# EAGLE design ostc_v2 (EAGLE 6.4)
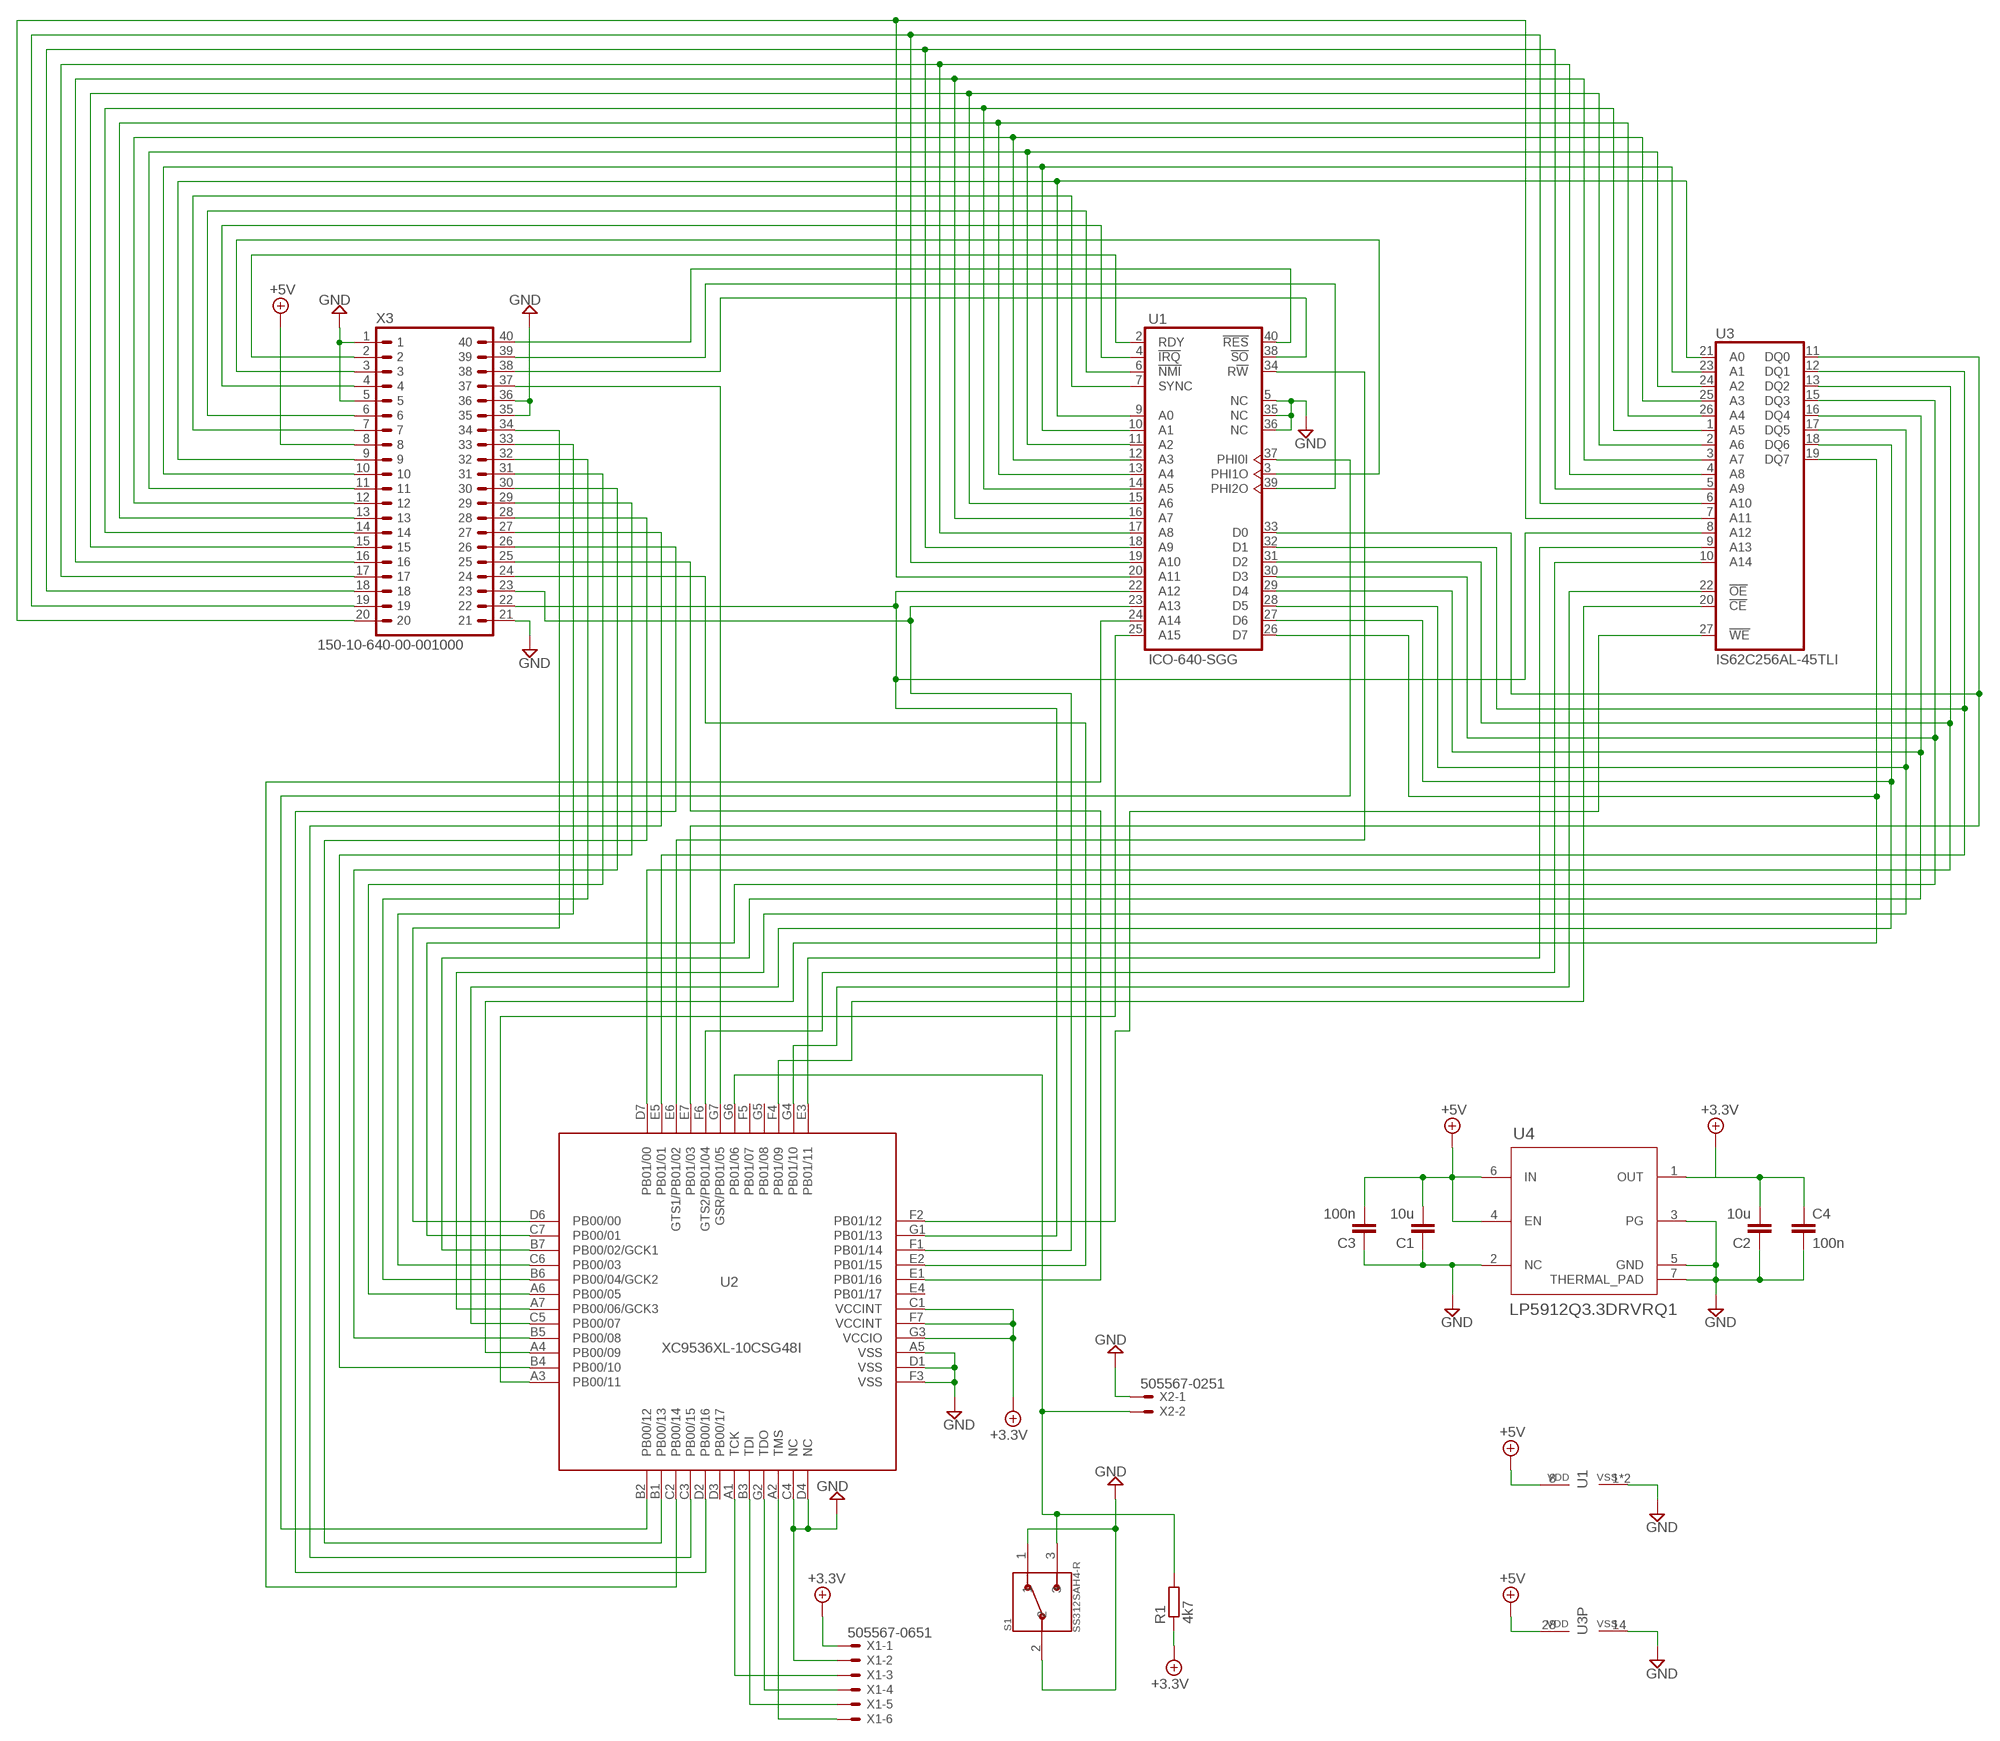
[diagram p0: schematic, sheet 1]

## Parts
C1  10u  C-EUC1206K  [C1206K]
C2  10u  C-EUC1206K  [C1206K]
C3  100n  C-EUC1206K  [C1206K]
C4  100n  C-EUC1206K  [C1206K]
R1  4k7  R-EU_R0805  [R0805]
S1  SS312SAH4-R  [SW_SS312SAH4-R]
U1  ICO-640-SGG  6502  [DIL40_LOWPROFILE]
U2  XC9536XL-10CSG48I  CX9536_CS48  [CSBGA48]
U3  IS62C256AL-45TLI  CY62256LL-ZC  [TSOP1-28]
U4  LP5912Q3.3DRVRQ1  LP5912-3.0DRVT  [DRV0006A-IPC_A]
X1  505567-0651  53261-06  [53261-06]
X2  505567-0251  53261-02  [53261-02]
X3  150-10-640-00-001000  DIL40  [DIL40]

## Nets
+3.3V: C2.2 C4.1 R1.1 U2.C1(VCCINT) U2.F7(VCCINT) U2.G3(VCCIO) U4.1(OUT) X1.1
+5V: C1.2 C3.2 U1.8(VDD) U3.28(VDD) U4.4(EN) U4.6(IN) X3.8
GND: C1.1 C2.1 C3.1 C4.2 S1.1 S1.2 U1.1(VSS) U1.5(NC) U1.21(VSS) U1.35(NC) U1.36(NC) U2.A5(VSS) U2.C4(NC) U2.D1(VSS) U2.D4(NC) U2.F3(VSS) U3.14(VSS) U4.2(NC) U4.3(PG) U4.5(GND) U4.7(THERMAL_PAD) X1.2 X2.1 X3.1 X3.5 X3.21 X3.35 X3.36
N$1: U1.2(RDY) X3.2
N$2: U1.3(PHI1O) X3.3
N$3: U1.4(!IRQ) X3.4
N$4: U1.6(!NMI) X3.6
N$5: U1.7(SYNC) X3.7
N$6: U1.9(A0) U3.21(A0) X3.9
N$7: U1.10(A1) U3.23(A1) X3.10
N$8: U1.11(A2) U3.24(A2) X3.11
N$9: U1.12(A3) U3.25(A3) X3.12
N$10: U1.13(A4) U3.26(A4) X3.13
N$11: U1.14(A5) U3.1(A5) X3.14
N$12: U1.15(A6) U3.2(A6) X3.15
N$13: U1.16(A7) U3.3(A7) X3.16
N$14: U1.17(A8) U3.4(A8) X3.17
N$15: U1.18(A9) U3.5(A9) X3.18
N$16: U1.19(A10) U3.6(A10) X3.19
N$17: U1.20(A11) U3.7(A11) X3.20
N$18: U2.E2(PB01/15) X3.24
N$19: U1.22(A12) U2.G1(PB01/13) U3.8(A12) X3.22
N$20: U1.23(A13) U2.F1(PB01/14) X3.23
N$21: U2.E1(PB01/16) X3.25
N$22: U2.D2(PB00/16) X3.26
N$23: U2.C3(PB00/15) X3.27
N$24: U2.B1(PB00/13) X3.28
N$25: U2.B4(PB00/10) X3.29
N$26: U2.B5(PB00/08) X3.30
N$27: U2.A6(PB00/05) X3.31
N$28: U2.B6(PB00/04/GCK2) X3.32
N$29: U2.C6(PB00/03) X3.33
N$30: U2.D6(PB00/00) X3.34
N$31: U2.G7(GSR/PB01/05) X3.37
N$32: U1.38(!SO) X3.38
N$33: U1.39(PHI2O) X3.39
N$34: U1.40(!RES) X3.40
N$35: U1.37(PHI0I) U2.B2(PB00/12)
N$36: U1.34(R!W) U2.E6(GTS1/PB01/02)
N$37: U1.33(D0) U2.E7(PB01/03) U3.11(DQ0)
N$38: U1.32(D1) U2.E5(PB01/01) U3.12(DQ1)
N$39: U1.31(D2) U2.D7(PB01/00) U3.13(DQ2)
N$40: U1.30(D3) U2.C7(PB00/01) U3.15(DQ3)
N$41: U1.29(D4) U2.B7(PB00/02/GCK1) U3.16(DQ4)
N$42: U1.28(D5) U2.A7(PB00/06/GCK3) U3.17(DQ5)
N$43: U1.27(D6) U2.C5(PB00/07) U3.18(DQ6)
N$44: U1.26(D7) U2.A4(PB00/09) U3.19(DQ7)
N$45: R1.2 S1.3 U2.G6(PB01/06) X2.2
N$47: U2.E3(PB01/11) U3.9(A13)
N$48: U2.F6(GTS2/PB01/04) U3.10(A14)
N$49: U2.G4(PB01/10) U3.22(!OE)
N$50: U2.F4(PB01/09) U3.20(!CE)
N$51: U2.F2(PB01/12) U3.27(!WE)
N$53: U1.25(A15) U2.A3(PB00/11)
N$54: U1.24(A14) U2.C2(PB00/14)
N$55: U2.A2(TMS) X1.6
N$56: U2.B3(TDI) X1.5
N$57: U2.G2(TDO) X1.4
N$58: U2.A1(TCK) X1.3
Unconnected: U2.D3(PB00/17) U2.E4(PB01/17) U2.F5(PB01/07) U2.G5(PB01/08)

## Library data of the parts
C1-C4 = resistor:C-EU: CAPACITOR, European symbol
R1 = resistor:R-EU_: RESISTOR, European symbol
S1 = SS312SAH4-R:SS312SAH4-R: Switch Slide ON None ON SPDT Side Slide 0.1A 28VAC 28VDC 0.4VA 10000Cycles Gull Wing SMD T/R; MANUFACTURER: NKK switches
U1 = 6502:6502: R6502 by Rockwell
U2 = xilinx-xc9:CX9536_CS48
U3 = memory-sram:CY62256LL-?*: 256K (32K x 8) CMOS-Static RAM Source: http://download.cypress.com.edgesuite.net/design_resources/datasheets/contents/cy62256_8.pdf
U4 = texas:LP5912-3.0DRVT; COPYRIGHT: Copyright (C) 2024 Ultra Librarian. All rights reserved.; MANUFACTURER_PART_NUMBER: LP5912-3.0DRVT; MFR_NAME: Texas Instruments; REFDES: RefDes; TYPE: TYPE
X1 = con-molex:53?-06: CONNECTOR wire to board 1.25 mm (.049 inch) pitch header; OC_FARNELL: 1125375; OC_NEWARK: unknown
X2 = con-molex:53?-02: CONNECTOR; OC_FARNELL: 1125373; OC_NEWARK: unknown
X3 = DIL-header:DIL40: DIL Header 40-pin

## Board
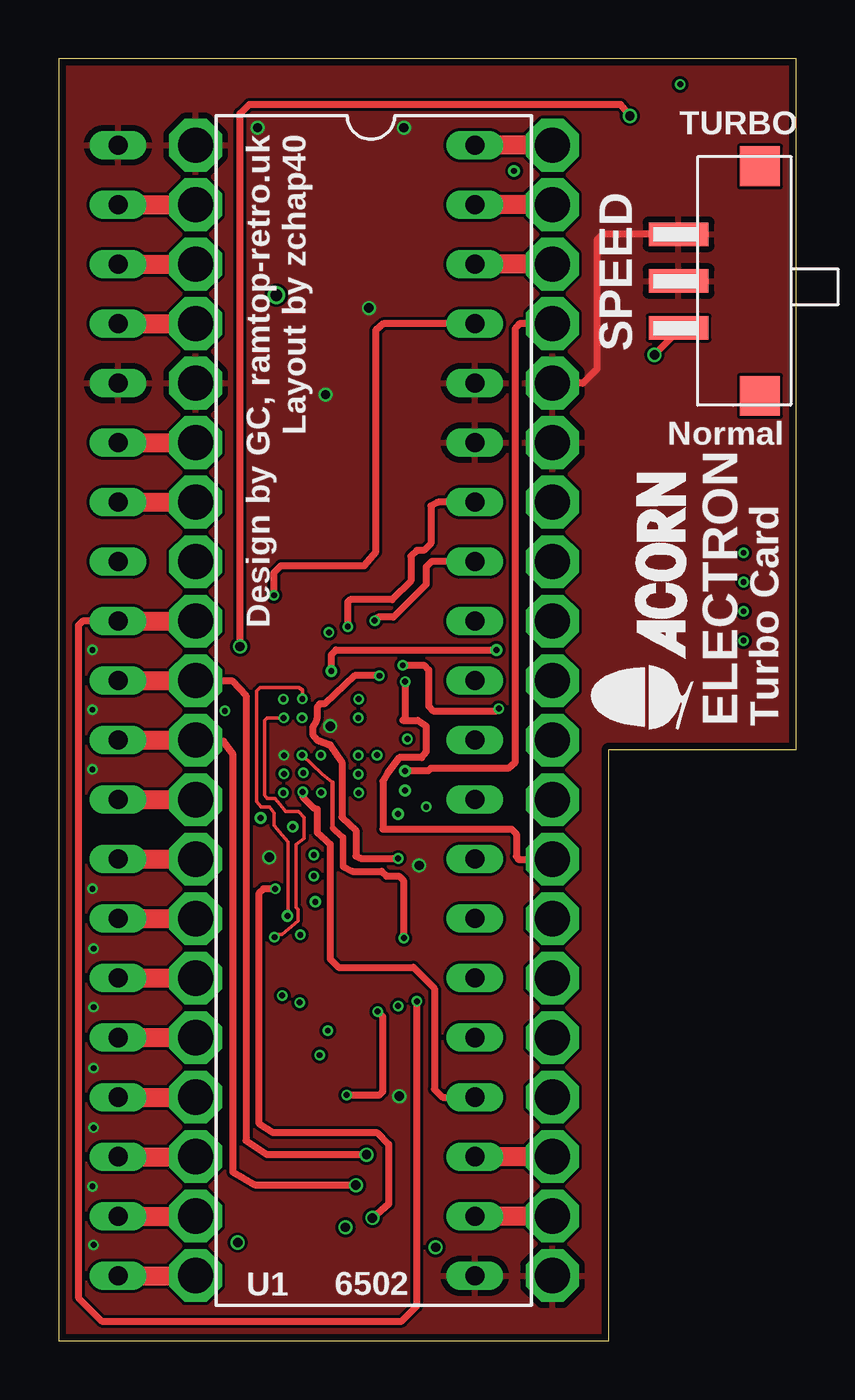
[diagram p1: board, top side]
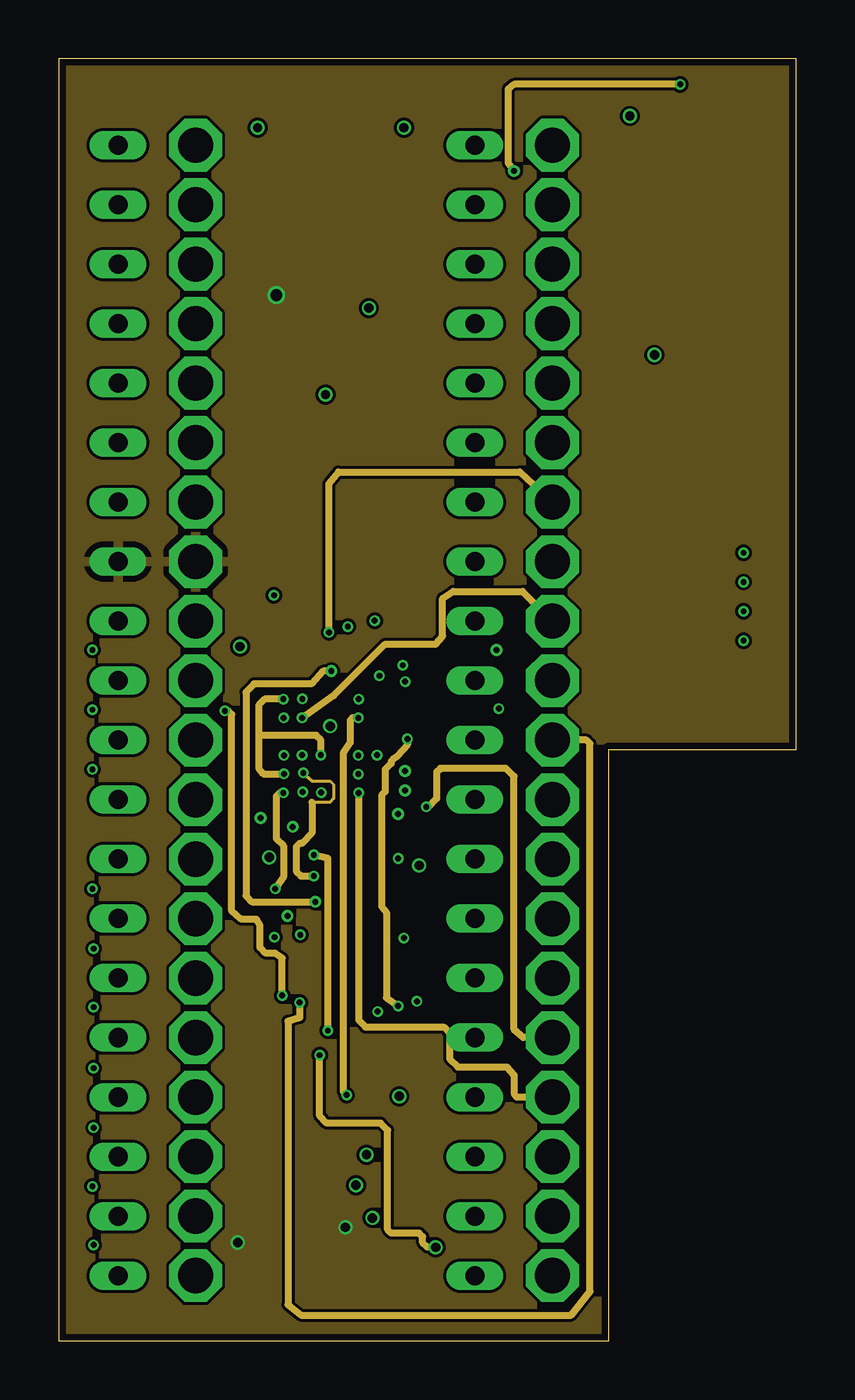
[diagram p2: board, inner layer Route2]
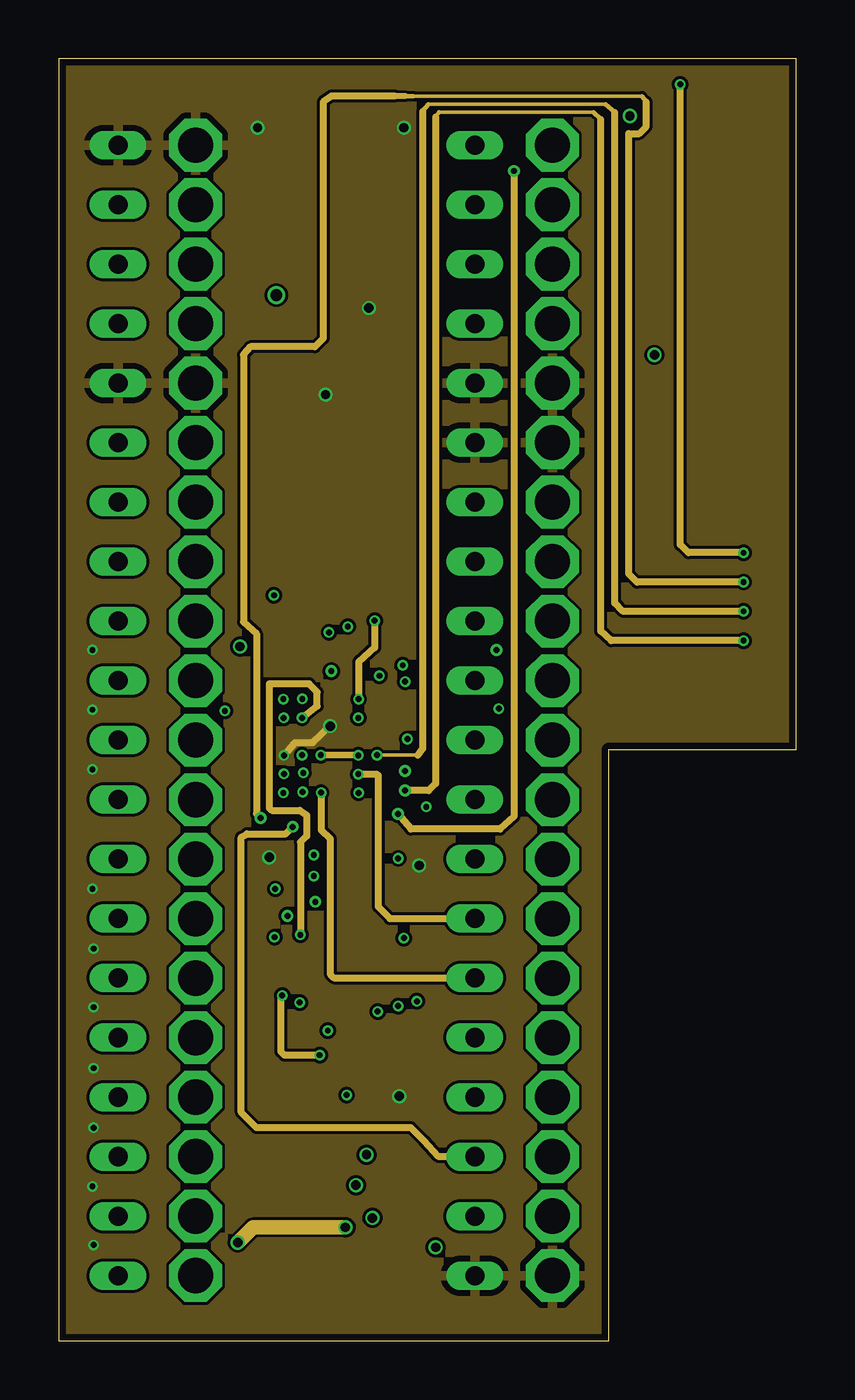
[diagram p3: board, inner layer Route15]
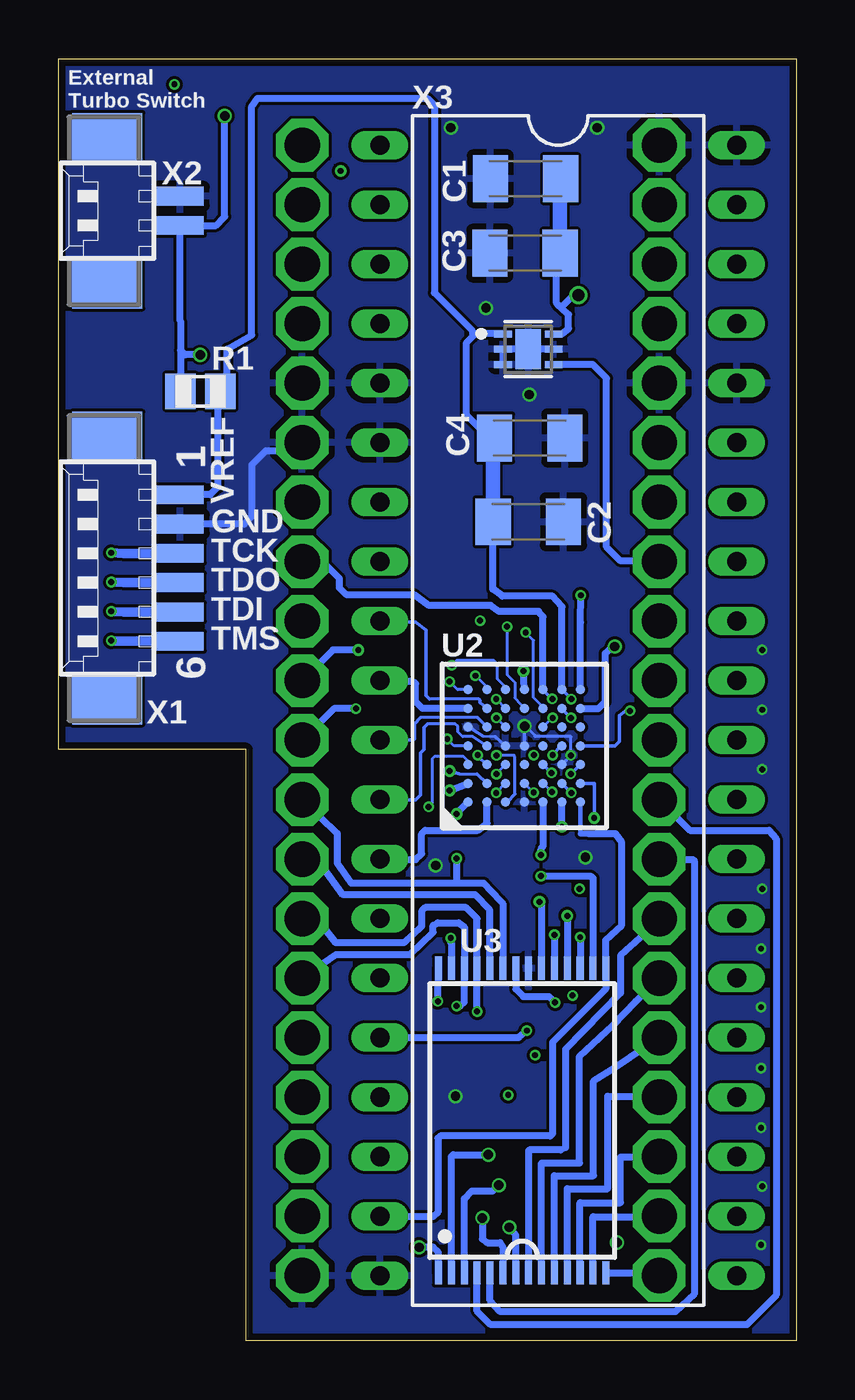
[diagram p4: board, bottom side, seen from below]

Size 31.5 x 54.75 mm. Coordinates in mm from the lower left corner, seen from the top.
Outline: 0,0 23.5,0 23.5,25.25 31.5,25.25 31.5,54.75 0,54.75 0,0
Copper layers (1+2*15+16): Top 0.035mm / dielectric 0.138mm / Route2 0.035mm / dielectric 1.13mm / Route15 0.035mm / dielectric 0.138mm / Bottom 0.035mm
Design rules "aisler_4_layer_complex *": minimum track width 0.125mm, minimum drill 0.1mm, track to track 0.125mm, track to pad 0.125mm, pad to pad 0.125mm, via to via 0.125mm, smd to smd 0mil, copper to edge 0.3mm, drill to drill 0.3mm, minimum pad ring 0.2mm, minimum via ring 0.1mm, stop-mask expansion 0mil, vias tented up to drill 0.3mm, thermal gap 10mil

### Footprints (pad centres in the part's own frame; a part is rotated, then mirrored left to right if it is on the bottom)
C1206K = smd 1.5 x 2: 1 -1.5,0; 2 1.5,0
R0805 = smd 1.3 x 1.5: 1 -0.85,0; 2 0.85,0
SW_SS312SAH4-R = smd 2.55 x 1: 1 1.525,-2; 2 1.525,0; 3 1.525,2 | smd 1.7 x 1.7: P$1 -1.95,-4.9; P$2 -1.95,4.9
DIL40_LOWPROFILE = drill 1.5 octagon: 1 -24.13,-7.62; 2 -21.59,-7.62; 3 -19.05,-7.62; 4 -16.51,-7.62; 5 -13.97,-7.62; 6 -11.43,-7.62; 7 -8.89,-7.62; 8 -6.35,-7.62; 9 -3.81,-7.62; 10 -1.27,-7.62; 11 1.27,-7.62; 12 3.81,-7.62; 13 6.35,-7.62; 14 8.89,-7.62; 15 11.43,-7.62; 16 13.97,-7.62; 17 16.51,-7.62; 18 19.05,-7.62; 19 21.59,-7.62; 20 24.13,-7.62; 21 24.13,7.62; 22 21.59,7.62; 23 19.05,7.62; 24 16.51,7.62; 25 13.97,7.62; 26 11.43,7.62; 27 8.89,7.62; 28 6.35,7.62; 29 3.81,7.62; 30 1.27,7.62; 31 -1.27,7.62; 32 -3.81,7.62; 33 -6.35,7.62; 34 -8.89,7.62; 35 -11.43,7.62; 36 -13.97,7.62; 37 -16.51,7.62; 38 -19.05,7.62; 39 -21.59,7.62; 40 -24.13,7.62
CSBGA48 = smd 0.4 x 0.4: A1 -2,2.8; A2 -1.2,2.8; A3 -0.4,2.8; A4 0.4,2.8; A5 1.2,2.8; A6 2,2.8; A7 2.8,2.8; B1 -2,2; B2 -1.2,2; B3 -0.4,2; B4 0.4,2; B5 1.2,2; B6 2,2; B7 2.8,2; C1 -2,1.2; C2 -1.2,1.2; C3 -0.4,1.2; C4 0.4,1.2; C5 1.2,1.2; C6 2,1.2; C7 2.8,1.2; D1 -2,0.4; D2 -1.2,0.4; D3 -0.4,0.4; D4 0.4,0.4; D6 2,0.4; D7 2.8,0.4; E1 -2,-0.4; E2 -1.2,-0.4; E3 -0.4,-0.4; E4 0.4,-0.4; E5 1.2,-0.4; E6 2,-0.4; E7 2.8,-0.4; F1 -2,-1.2; F2 -1.2,-1.2; F3 -0.4,-1.2; F4 0.4,-1.2; F5 1.2,-1.2; F6 2,-1.2; F7 2.8,-1.2; G1 -2,-2; G2 -1.2,-2; G3 -0.4,-2; G4 0.4,-2; G5 1.2,-2; G6 2,-2; G7 2.8,-2
TSOP1-28 = smd 1 x 0.3: 1 -6.5,-0.275; 2 -6.5,-0.825; 3 -6.5,-1.375; 4 -6.5,-1.925; 5 -6.5,-2.475; 6 -6.5,-3.025; 7 -6.5,-3.575; 8 6.5,-3.575; 9 6.5,-3.025; 10 6.5,-2.475; 11 6.5,-1.925; 12 6.5,-1.375; 13 6.5,-0.825; 14 6.5,-0.275; 15 6.5,0.275; 16 6.5,0.825; 17 6.5,1.375; 18 6.5,1.925; 19 6.5,2.475; 20 6.5,3.025; 21 6.5,3.575; 22 -6.5,3.575; 23 -6.5,3.025; 24 -6.5,2.475; 25 -6.5,1.925; 26 -6.5,1.375; 27 -6.5,0.825; 28 -6.5,0.275
DRV0006A-IPC_A = smd 0.756 x 0.292: 1 -1.078,0.65; 2 -1.078,0; 3 -1.078,-0.65; 4 1.078,-0.65; 5 1.078,0; 6 1.078,0.65 | smd 1.1 x 1.7: 7 0,0
53261-06 = smd 0.8 x 2: 1 3.125,-2.5; 2 1.875,-2.5; 3 0.625,-2.5; 4 -0.625,-2.5; 5 -1.875,-2.5; 6 -3.125,-2.5 | smd 2.1 x 3: S1 5.625,0.625; S2 -5.625,0.625
53261-02 = smd 0.8 x 2: 1 0.625,-2.5; 2 -0.625,-2.5 | smd 2.1 x 3: S1 3.125,0.625; S2 -3.125,0.625
DIL40 = drill 0.813 long: 1 -24.13,-7.62; 2 -21.59,-7.62; 3 -19.05,-7.62; 4 -16.51,-7.62; 5 -13.97,-7.62; 6 -11.43,-7.62; 7 -8.89,-7.62; 8 -6.35,-7.62; 9 -3.81,-7.62; 10 -1.27,-7.62; 11 1.27,-7.62; 12 3.81,-7.62; 13 6.35,-7.62; 14 8.89,-7.62; 15 11.43,-7.62; 16 13.97,-7.62; 17 16.51,-7.62; 18 19.05,-7.62; 19 21.59,-7.62; 20 24.13,-7.62; 21 24.13,7.62; 22 21.59,7.62; 23 19.05,7.62; 24 16.51,7.62; 25 13.97,7.62; 26 11.43,7.62; 27 8.89,7.62; 28 6.35,7.62; 29 3.81,7.62; 30 1.27,7.62; 31 -1.27,7.62; 32 -3.81,7.62; 33 -6.35,7.62; 34 -8.89,7.62; 35 -11.43,7.62; 36 -13.97,7.62; 37 -16.51,7.62; 38 -19.05,7.62; 39 -21.59,7.62; 40 -24.13,7.62

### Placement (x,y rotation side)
C1  11.56,49.62 0 bottom
C2  11.44,34.97 180 bottom
C3  11.58,46.44 0 bottom
C4  11.38,38.55 0 bottom
R1  25.44,40.54 180 bottom
S1  28,45.25 180 top
U1  13.47,26.92 270 top
U2  11.21,25.01 90 bottom
U3  11.7,9.41 90 bottom
U4  11.44,42.34 0 bottom
X1  28.8,33 90 bottom
X2  28.8,48.25 90 bottom
X3  10.16,26.92 270 top

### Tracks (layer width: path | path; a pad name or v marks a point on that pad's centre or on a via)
+3.3V  (via drill 0.25)
  Route2 0.305: v11.2,25.01 11.2,25.65 11,25.85 8.55,25.85 | 8.55,25.85 8.55,24.45 8.74,24.21 v9.62,24.21 | v9.6,27.4 8.8,27.4 8.55,27.15 8.55,25.85
  Route15 0.305: v12.8,25 v11.2,25.01
  Bottom 0.125: 12.01,23.35 12.01,24.95 12.05,25 v12.8,25
  Bottom 0.15: U2.G3 9.57,24.25 v9.62,24.21 | U2.F7 10.01,27.76 9.96,27.76 v9.6,27.4 | U2.C1 12.34,23.01 12.01,23.35
  Bottom 0.305: U4.1 13.7,43 13.82,42.88 | 13.82,42.88 14.1,42.6 14.1,39.55 13.1,38.55 C4.1 | X1.1 25.02,36.12 24.7,36.45 24.7,40.43 R1.1 24.65,40.6 24.3,40.6 24.3,42.35 23.25,42.95 23.25,52.7 23,53.05 15.75,53.05 15.45,52.75 15.45,44.75 13.82,43.12 13.82,42.88 | U2.F7 10,31.35 10.4,31.8 12.55,31.8 12.95,32.1 C2.2
  Bottom 0.61: C2.2 12.94,38.49 C4.1
+5V  (via drill 0.4, 0.5)
  Route15 0.61: v12.25,4.85 8.3,4.85 v7.65,4.2
  Bottom 0.305: U1.8 5.88,33.3 7.5,33.3 8.1,33.9 8.1,41.1 8.69,41.69 U4.4 | U4.6 10,43 9.73,43.23 9.73,43.83 10.05,44.11 | C3.2 10.25,46.16 10.25,44.35 10.18,44.23 10.05,44.11 | U3.28 11.97,4.51 v12.25,4.85 | v9.3,44.65 9.51,44.65 10.05,44.11
  Bottom 0.61: C3.2 10.08,49.6 C1.2
  pour Route2: 0,0 0,54.75 31.5,54.75 31.5,25.25 23.5,25.25 23.5,0
GND  (via drill 0.25 pad 0.45, 0.4, 0.4 pad 0.45)
  Top 0.305: S1.1 23.25,47.25 23,47 23,41.5 22.39,40.89 U1.36
  Route15 0.305: v9.62,25 9.62,25.02 10.1,25.55 10.85,25.55 v11.6,26.25
  Bottom 0.125: 13.78,26.09 13.38,25.82 12.86,25.81 | v9.62,25 9.61,25.8 11.15,25.8 11.15,25.85 11.55,26.25 v11.6,26.25
  Bottom 0.15: 12.38,25.41 U2.C4 12.86,25.81 | U2.A5 13.88,26.21 13.78,26.09 | U2.D4 v11.6,26.25 | U2.F3 v9.62,25
  Bottom 0.305: 13,49.68 C1.1 12.95,49.51 | U4.3 U4.2 11.56,42.34 11.5,42.4 U4.7 U4.5 | 10.4,38.62 C4.2 10.35,38.52 | U1.35 21.44,38 22.65,38 23.25,37.4 23.25,35.2 23.57,34.88 X1.2
  other vias: 9,20.65 1.45,29.5 1.45,26.95 1.45,24.4 1.45,19.3 1.5,16.75 1.5,14.25 1.5,11.65 1.5,9.1 1.45,6.6 1.5,4.1 15.4,20.3 14.55,10.45 11.4,40.4 13.25,44.1 14.75,51.8 8.5,51.8
  pour Route15: 0,54.75 31.5,54.75 31.5,25.25 23.5,25.25 23.5,0 0,0
  pour Bottom: 0,54.75 31.5,54.75 31.5,25.25 23.5,25.25 23.5,0 0,0
  pour Top: 0,54.75 31.5,54.75 31.5,25.25 23.5,25.25 23.5,0 0,0
N$1
  Top 0.813: X3.2 U1.2
N$2
  Top 0.813: X3.3 U1.3
N$3
  Top 0.813: X3.4 U1.4
N$4
  Top 0.813: X3.6 U1.6
N$5
  Top 0.813: X3.7 U1.7
N$6  (via drill 0.25)
  Top 0.305: U1.9 1.03,30.73 0.85,30.55 0.85,1.85 1.85,0.85 14.65,0.85 15.3,1.5 v15.3,14.5
  Top 0.813: X3.9 U1.9
  Bottom 0.305: v15.3,14.5 15.3,14.7 15.29,15.9 U3.21
N$7  (via drill 0.4)
  Top 0.305: U1.10 7.41,28.19 8,27.55 8,8.55 8.9,7.95 v13.15,7.95
  Top 0.813: X3.10 U1.10
  Bottom 0.305: U3.23 14.72,7.88 14.65,7.95 v13.15,7.95
N$8  (via drill 0.4)
  Top 0.305: v12.7,6.65 8.4,6.65 7.45,7.2 7.45,25.05 7.05,25.6 5.9,25.6 U1.11
  Top 0.813: X3.11 U1.11
  Bottom 0.305: U3.24 14.18,6.08 13.85,6.4 12.95,6.4 v12.7,6.65
N$9
  Top 0.813: X3.12 U1.12
  Bottom 0.305: U1.12 4.54,21.8 1.15,21.8 0.85,21.45 0.85,1.95 2.1,0.7 13.05,0.7 13.62,1.27 U3.25
N$10
  Top 0.813: X3.13 U1.13
  Bottom 0.305: U1.13 5.83,20.55 4.4,20.55 4.35,20.5 4.35,2 5.15,1.25 12.65,1.25 13.07,1.73 U3.26
N$11
  Top 0.813: X3.14 U1.14
  Bottom 0.305: U1.14 5.85,17.95 7.5,16.45 7.5,14.85 9.85,12.45 9.85,8.25 10.05,8.15 11.4,8.15 11.43,8.12 U3.1
N$12
  Top 0.813: X3.15 U1.15
  Bottom 0.305: U3.2 10.88,7.6 9.25,7.6 9.25,12.15 7.8,13.5 6.85,14.5 5.85,15.45 U1.15
N$13
  Top 0.813: X3.16 U1.16
  Bottom 0.305: U3.3 10.33,7.05 8.65,7.05 8.65,11.1 7.7,11.7 U1.16
N$14
  Top 0.813: X3.17 U1.17
  Bottom 0.305: U3.4 9.77,6.46 9.77,6.5 8.05,6.5 8.05,10.45 5.85,10.45 U1.17
N$15
  Top 0.813: X3.18 U1.18
  Bottom 0.305: U3.5 9.23,5.9 7.5,5.9 7.5,7.85 5.85,7.85 U1.18
N$16
  Top 0.813: X3.19 U1.19
  Bottom 0.305: U3.6 8.68,5.3 5.85,5.3 U1.19
N$17
  Top 0.813: X3.20 U1.20
  Bottom 0.305: U3.7 5.85,2.91
  Bottom 0.406: 5.85,2.91 U1.20
N$18  (via drill 0.25 pad 0.45)
  Top 0.305: v10.43,23.44 10.43,23.23 10.9,22.75 11.05,22.7 11.05,21.7 11.4,21.4 11.6,21.2 11.6,16.3 11.95,15.95 15.15,15.95 16.05,15.05 16.05,10.75 16.4,10.4 X3.24
  Bottom 0.125: U2.E2 10.8,23.81 v10.43,23.44
N$19
  Top 0.813: U1.22 X3.22
  Bottom 0.2: 9.21,21.65 U2.G1
  Bottom 0.25: 8.85,21.65 9.21,21.65
  Bottom 0.275: 8.55,21.65 8.85,21.65
  Bottom 0.305: U3.8 8.13,17.12 7.45,17.75 7.45,21.3 7.7,21.65 8.55,21.65 | U3.8 | U3.8 8.13,15.02 10.4,12.75 10.4,8.85 10.5,8.75 15.2,8.75 15.3,8.65 15.3,5.5 15.5,5.3 17.75,5.3 X3.22
N$20  (via drill 0.25 pad 0.5)
  Top 0.813: U1.23 X3.23
  Route15 0.305: X3.23 16.23,7.87 15.6,8.55 15.05,9.1 8.45,9.1 7.8,9.75 7.8,21.5 8.05,21.65 9.7,21.65 v10,21.95
  Bottom 0.305: v10,21.95 U2.F1
N$21  (via drill 0.25 pad 0.45)
  Route2 0.305: v11.5,13.25 11.5,20.6 v10.9,20.75
  Bottom 0.305: X3.25 11.85,12.95 v11.5,13.25 | v10.9,20.75 10.9,21 10.8,21.15 U2.E1
N$22  (via drill 0.25 pad 0.45)
  Route15 0.305: v11.21,23.41 11.21,21.81 11.6,21.45 11.6,15.65 11.75,15.5 X3.26
  Bottom 0.125: U2.D2 v11.21,23.41
N$23  (via drill 0.25 pad 0.45)
  Route15 0.305: v12.8,24.2 13.6,24.2 13.65,24.15 13.65,18.55 14.15,18.04 X3.27
  Bottom 0.125: U2.C3 12.44,24.61 v12.8,24.2
N$24
  Bottom 0.305: X3.28 17.76,20.55 16.25,20.55 16,20.8 16,21.65 15.85,21.8 13.6,21.8 13.2,22.1 U2.B1
N$25
  Bottom 0.125: U2.B4 13.8,25.8 14.25,25.8 14.45,26 14.45,26.25 14.55,26.35 15.75,26.35
  Bottom 0.15: 15.75,26.35 15.9,26.2 15.9,25.25 16.05,25.1 16.05,23.3 16.25,23.1 X3.29
N$26
  Bottom 0.125: 13.6,26.61 16.05,26.61
  Bottom 0.15: U2.B5 13.6,26.61 | 16.05,26.61 16.3,26.35 16.3,25.7 16.35,25.65 X3.30
N$27
  Bottom 0.305: U2.A6 15.96,27.01 16.25,27.3 16.25,28.05 16.35,28.15 17.74,28.15 X3.31
N$28
  Bottom 0.125: 13.5,27.35 13.55,27.41 15.66,27.41
  Bottom 0.15: U2.B6 13.5,27.25 13.5,27.35 | 15.66,27.41 15.8,27.55 15.8,30.35 16.25,30.7 17.75,30.7 X3.32
N$29  (via drill 0.25 pad 0.45)
  Top 0.305: X3.33 15.92,33.27 15.7,33.05 15.7,32.3 14.3,30.9 13.65,30.9 v13.5,30.75
  Route15 0.305: v13.5,30.75 13.5,29.6 12.81,28.99 v12.81,27.4
  Bottom 0.125: v12.81,27.4 v12.8,27.4 U2.C6
N$30  (via drill 0.25 pad 0.45)
  Top 0.305: X3.34 16.21,35.81 15.9,35.65 15.9,34.05 15.6,33.75 15.3,33.75 15.05,33.5 15.05,32.45 14.25,31.65 12.45,31.65 12.35,31.55 v12.35,30.5
  Bottom 0.125: v12.35,30.5 12.35,28.45 12.01,28.11 12.01,27.45 U2.D6
N$31  (via drill 0.25 pad 0.45)
  Top 0.305: v9.2,31.84 9.2,32.8 9.5,33.1 13.05,33.1 13.55,33.7 13.55,43.15 13.9,43.45 17.76,43.45 X3.37
  Bottom 0.305: U2.G7 9.21,30.69 v9.2,31.84
N$32
  Top 0.813: U1.38 X3.38
N$33
  Top 0.813: U1.39 X3.39
N$34
  Top 0.813: U1.40 X3.40
N$35  (via drill 0.25 pad 0.5)
  Top 0.305: U1.37 19.68,43.43 19.5,43.2 19.5,24.7 19.2,24.45 15.9,24.45 15.79,24.34 v14.8,24.34
  Bottom 0.125: 14.38,24.21 13.62,24.21
  Bottom 0.15: v14.8,24.34 14.8,24.25 14.5,24.25 14.38,24.21 | 13.62,24.21 U2.B2
N$36  (via drill 0.25 pad 0.45)
  Route2 0.305: v11.55,30.25 11.55,36.6 11.95,37.1 19.7,37.1 U1.34
  Bottom 0.125: U2.E6 10.81,27.06 11.21,27.46 11.21,29.91 v11.55,30.25
N$37  (via drill 0.25 pad 0.45, 0.25 pad 0.5)
  Top 0.15: v10.41,27.41 10.41,27.79 10.25,27.9 8.6,27.9 8.46,27.75 8.46,23.04 8.65,22.8 9.01,22.8 9.2,22.55 9.2,22 9.55,21.6 9.8,21.3 9.8,18.2 v9.78,18.15
  Bottom 0.15: U2.E7 10.81,27.76 v10.41,27.41 | 9.78,15.94 U3.11
  Bottom 0.305: U2.E7 10.81,30.91 11,31.15 12.7,31.15 13.05,31.4 15.7,31.4 16.3,31.85 19.2,31.85 19.5,32.15 19.5,32.55 20.22,33.27 U1.33 | v9.78,18.15 9.78,15.94
N$38  (via drill 0.25 pad 0.45)
  Route2 0.305: U1.32 19.82,32 16.85,32 16.4,31.7 16.4,30.1 16.1,29.75 13.95,29.75 11.75,27.55 v10.4,26.6
  Route15 0.305: v10.32,17.34 10.32,21.3 10.6,21.55 10.6,22.45 10.3,22.65 9.1,22.65 9,22.75 9,28.05 10.7,28.05 11.05,27.7 11.05,27.1 v10.4,26.6
  Bottom 0.125: U2.E5 10.81,26.24 v10.4,26.6
  Bottom 0.305: v10.32,17.34 U3.12
N$39  (via drill 0.25 pad 0.5)
  Top 0.305: v11.65,28.6 11.65,29.3 11.85,29.5 v18.7,29.5
  Route2 0.305: v11.65,28.6 11.3,28.6 10.8,28.05 8.35,28.05 8,27.7 8,19 8.25,18.75 v10.96,18.75
  Bottom 0.15: U2.D7 11.61,28.59 v11.65,28.6
  Bottom 0.305: U2.D7 v11.65,28.6 | v18.7,29.5 19.78,29.5 U1.31 | v10.96,18.75 10.88,18.61 U3.13
N$40  (via drill 0.25 pad 0.45)
  Top 0.305: v14.7,28.85 15.6,28.85 15.8,28.65 15.8,27.1 16,26.9 18.7,26.9 v18.8,27
  Route2 0.305: v10.3,14.45 10.3,13.8 9.8,13.65 9.8,1.55 10.35,1.1 21.9,1.1 22.7,2.1 22.7,25.5 22.55,25.65 U1.30
  Bottom 0.125: U2.C7 12.41,27.91 12.75,28.25 12.75,28.9 12.9,29.05 14.5,29.05 v14.7,28.85
  Bottom 0.305: v18.8,27 19.74,27 U1.30 | U3.15 11.97,15.03 11.65,14.7 10.55,14.7 v10.3,14.45
N$41  (via drill 0.25 pad 0.45)
  Top 0.305: v13.7,28.4 12.65,28.4 11.35,27.2 11.15,27.2 11.05,27.05 11.05,26.61 10.99,26.44 10.85,26.2 10.85,25.9 11.05,25.65 11.6,25.45 12.1,24.7 12.1,22.35 12.7,21.8 12.7,20.7 12.9,20.6 v14.5,20.6
  Bottom 0.125: U2.B7 13.21,27.91 v13.7,28.4
  Bottom 0.305: U1.29 19.6,21.67 19.6,20.4 19,19.55 14.4,19.55 | 14.4,19.55 13.35,19.55 12.65,18.8 12.53,18.68 U3.16 | v14.5,20.6 14.5,19.6 14.4,19.55
N$42  (via drill 0.25 pad 0.45)
  Top 0.305: v14.8,28.15 14.8,26.6 14.7,26.5 15.35,26.5 15.7,26.25 15.7,25.15 15.5,24.9 14.55,24.9 14.05,24.25 13.85,23.9 13.85,21.85 19.35,21.85 19.55,21.65 19.55,20.7 19.64,20.56 20.52,20.56 20.6,20.57 U1.28
  Bottom 0.125: U2.A7 14.46,27.81 v14.8,28.15
  Bottom 0.305: U3.17 13.08,15.98 13.08,18.4 13.7,19.05 19.35,19.05 20.47,20.57 U1.28
N$43  (via drill 0.25 pad 0.45)
  Top 0.305: v12.3,10.5 13.7,10.5 13.85,10.65 13.85,13.84 v13.62,14.06
  Route2 0.305: v12.8,26.6 12.55,26.6 12.45,26.5 12.45,25.55 12.15,25.1 12.15,10.65 v12.3,10.5
  Bottom 0.125: U2.C5 v12.8,26.6
  Bottom 0.305: U1.27 20.47,18.03 19.65,17 16.75,17 16,17.7 16,18.35 15.85,18.5 14.1,18.5 13.63,18.03 13.63,15.94 U3.18 v13.62,14.06
N$44  (via drill 0.25 pad 0.45)
  Route2 0.305: v14.9,25.7 14.9,25.45 14.45,24.95 14.3,24.85 14.2,24.75 14.2,24.65 13.95,24.4 13.95,23.45 13.8,23.3 13.8,18.55 14,18.3 14,14.65 v14.5,14.3
  Bottom 0.125: U2.A4 14.61,25.41 v14.9,25.7
  Bottom 0.305: U1.26 19.65,16.5 16.5,16.5 15.5,17.45 15.5,17.75 15.3,17.85 14.4,17.85 14.18,17.68 U3.19 14.18,14.47 14.35,14.3 v14.5,14.3
N$45  (via drill 0.4)
  Top 0.305: v7.75,29.65 7.75,52.4 8.15,52.8 24,52.8 v24.4,52.3 | S1.3 26.48,43.12 v25.45,42.1
  Bottom 0.305: U2.G6 8.45,27 8.15,27.3 8.15,29.35 7.85,29.65 v7.75,29.65 | v24.4,52.3 24.4,48 24.77,47.62 X2.2 26.3,43.55 26.29,43.55 26.29,42.3 | 26.29,42.3 R1.2 | v25.45,42.1 26.09,42.1 26.29,42.3
N$47  (via drill 0.25 pad 0.45)
  Route2 0.125: 10.82,23.9 11.6,23.9 11.75,23.75 11.75,23.15 11.6,23 10.82,23
  Route2 0.15: v10.45,24.25 10.45,24.24 10.82,23.9
  Route2 0.305: 10.82,23 10.82,21.69 10.4,21.25 10.3,21.25 10.15,21.1 10.15,20.05 10.35,19.85 v10.9,19.85
  Bottom 0.15: U2.E3 v10.45,24.25
  Bottom 0.305: v10.9,19.85 8.78,19.85 8.68,19.75 U3.9
N$48  (via drill 0.25 pad 0.45)
  Top 0.15: v9.61,26.6 8.9,26.6 8.8,26.5 8.8,23.3 8.9,23.15 9.25,23.15 9.55,22.8 9.7,22.6 10.25,22.6 10.47,22.35 10.47,21.46 10.15,21.2 10.15,18.5 10.22,18.43 10.22,17.94 9.55,17.35 9.35,17.35 v9.22,17.24
  Bottom 0.15: U2.F6 10.01,26.99 v9.61,26.6
  Bottom 0.305: v9.22,17.24 U3.10
N$49  (via drill 0.25, 0.4)
  Route2 0.305: v16.1,4 15.75,4 15.55,4.2 15.55,4.45 15.4,4.6 14.2,4.6 14.05,4.75 14.05,9 13.75,9.3 11.45,9.3 11.15,9.6 v11.15,12.2 | v9.55,14.75 9.55,16.35 9.25,16.55 8.85,16.55 8.6,16.8 8.6,17.75 8.45,18 7.8,18 7.4,18.35 7.4,26.75 7.25,26.9 v7.1,26.9
  Route15 0.305: v11.15,12.2 9.65,12.2 9.5,12.35 9.5,14.7 v9.55,14.75
  Bottom 0.15: 9.21,25.46 U2.G4 7.75,25.4 7.55,25.6 7.55,26.7 7.3,26.9 v7.1,26.9
  Bottom 0.305: U3.22 15.28,3.77 15.5,4 v16.1,4
N$50  (via drill 0.25 pad 0.45)
  Top 0.15: v10.4,25.01 11.26,24.2 11.7,23.85
  Top 0.2: 11.7,23.85 11.7,22.45 11.7,21.9
  Top 0.225: 11.7,21.9 11.8,21.8
  Top 0.25: 11.8,21.8 12.15,21.5
  Top 0.275: 12.15,21.5 12.15,20.25
  Top 0.29: 12.15,20.25 12.55,20.05
  Top 0.305: 12.55,20.05 13.8,20.05 14,19.85 14.54,19.85 14.72,19.66 14.72,17.23 v14.75,17.2
  Bottom 0.15: U2.F4 10.04,25.41 v10.4,25.01
  Bottom 0.305: v14.75,17.2 14.75,17.01 14.72,16.99 U3.20
N$51  (via drill 0.25 pad 0.45, 0.4 pad 0.45)
  Top 0.305: v9.25,19.3 8.75,19.3 8.55,19.1 8.55,9.3 9.15,8.9 13.6,8.9 14.1,8.4 14.1,5.85 v13.4,5.25
  Route2 0.305: v9.6,23.4 9.45,23.4 9.3,23.25 9.3,21.45 9.6,21.15 9.6,19.8 v9.25,19.3
  Bottom 0.15: U2.F2 v9.6,23.4
  Bottom 0.305: v13.4,5.25 13.4,4.35 13.2,4.2 12.65,4.2 12.53,4 U3.27
N$53  (via drill 0.25 pad 0.45)
  Route2 0.305: U1.25 19.85,12.95 19.45,13.3 19.45,24.1 19.1,24.45 16.3,24.45 16.15,24.3 16.15,23.15 15.8,22.8 v15.7,22.8
  Bottom 0.125: U2.A3 14.01,24.76 14.2,24.95 15.45,24.95 15.55,24.85 15.55,22.95 v15.7,22.8
N$54  (via drill 0.25 pad 0.45)
  Route2 0.305: v12.81,23.4 12.81,13.7 13.1,13.4 16.45,13.4 16.7,13.15 16.7,12.05 17.05,11.7 19.15,11.7 19.45,11.35 19.45,10.55 19.56,10.41 U1.24
  Bottom 0.125: U2.C2 12.44,23.81 v12.81,23.4
N$55  (via drill 0.25, 0.25 pad 0.5)
  Route15 0.15: 22.85,52.45 16.25,52.45
  Route15 0.2: 23.15,52.15 22.85,52.45 | 16.25,52.45 16.1,52.25
  Route15 0.305: v29.25,29.9 23.6,29.9 23.15,30.3 23.15,52.15 | 16.1,52.25 16.1,23.8 15.8,23.5 v14.8,23.5
  Bottom 0.305: v14.8,23.5 U2.A2
  Bottom 0.406: X1.6 29.25,29.88 v29.25,29.9
N$56  (via drill 0.25, 0.25 pad 0.45)
  Route15 0.15: 23.35,52.8 15.8,52.8 | 15.35,25.01 v13.6,25.01
  Route15 0.2: 23.75,52.45 23.35,52.8 | 15.8,52.8 15.55,52.5
  Route15 0.305: v29.25,31.15 24.1,31.15 23.75,31.5 23.75,52.45 | 15.55,52.5 15.55,25.29 15.35,25.01
  Bottom 0.15: v13.6,25.01 13.6,24.96 U2.B3
  Bottom 0.406: X1.5 28.73,31.12 v29.25,31.15
N$57  (via drill 0.25, 0.25 pad 0.5)
  Route15 0.15: 24.9,53.15 15.15,53.15
  Route15 0.2: 25.1,52.9 24.9,53.15 | 15.15,53.15 14.8,53.15
  Route15 0.25: 14.8,53.15 14.35,53.15
  Route15 0.305: v29.25,32.4 24.7,32.4 24.35,32.75 24.35,51.55 24.8,51.55 25.1,51.85 25.1,52.9 | 14.35,53.15 11.65,53.15 11.3,52.9 11.3,42.8 10.95,42.45 8.2,42.45 7.9,42.1 7.9,30.7 8.45,30.2 8.45,22.51 v8.62,22.32
  Bottom 0.15: v8.62,22.32 8.62,23.8 U2.G2
  Bottom 0.406: X1.4 28.73,32.38 v29.25,32.4
N$58  (via drill 0.25, 0.25 pad 0.5)
  Route2 0.305: v26.55,53.65 19.45,53.65 19.2,53.45 19.2,50.3 v19.45,49.95
  Route15 0.305: v29.25,33.65 26.9,33.65 26.55,34 v26.55,53.65 | v19.45,49.95 19.45,22.4 18.85,21.85 15.05,21.85 v14.5,22.5
  Bottom 0.15: v14.5,22.5 14.5,22.52
  Bottom 0.305: 14.5,22.52 U2.A1
  Bottom 0.406: X1.3 28.73,33.62 v29.25,33.65

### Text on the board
tNames: Design by GC, ramtop-retro.uk / Layout by zchap40 | TURBO | SPEED | Normal | ELECTRON | Turbo Card | 6502
bNames: X3 | External / Turbo Switch | X2 | 1 | VREF | GND | TCK | TDO | TDI | TMS | 6 | X1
